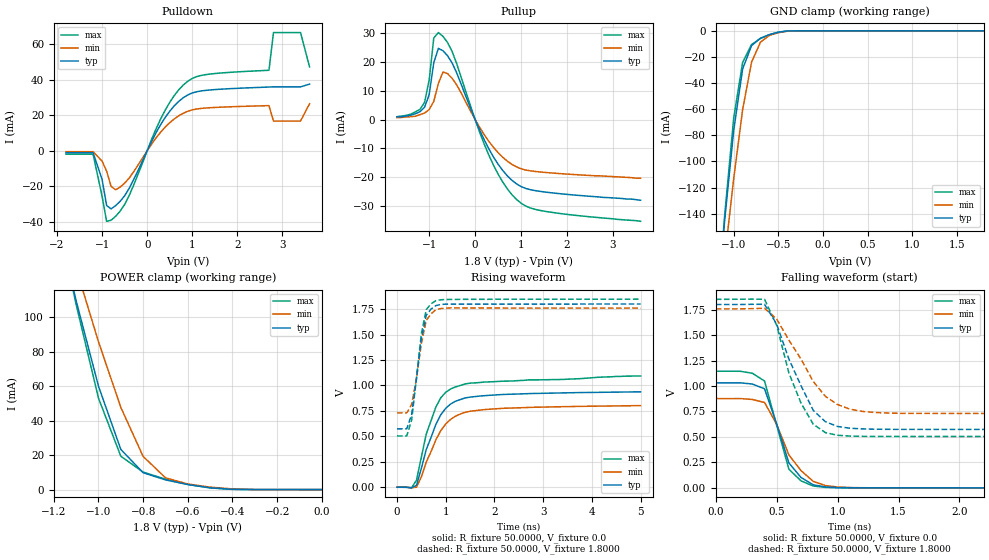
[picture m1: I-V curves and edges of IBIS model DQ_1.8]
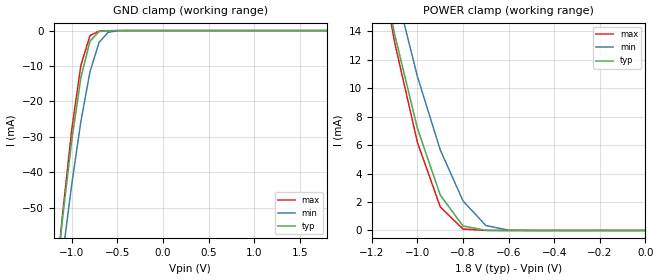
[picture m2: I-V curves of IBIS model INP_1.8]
|*** ISSI Synchronous Sram IBIS Model ***
[IBIS ver]	3.2
[File name]	is61nvvp204836165bga.ibs
[File Rev]	1.0
[Date]	May 13,2013
[Notes]
|--- Version History --------------------------------
|1.0: prelimiary
[Disclaimer]	This information is for modeling purpose only
		and is not guaranteed
[Copyright]	INTEGRATED SILICON SOLUTION, INC. 2011
[Component]	IS61NVVP204836_165BGA
[Manufacturer]	ISSI
[Package]
| variable   typ   min   max
R_pkg		100.34m			23.84m			218.59m
L_pkg		1.3400nH		0.3700nH		3.0300nH
C_pkg		41.410pF		0.4200pF		150.38pF
[Pin]  signal_name   model_name   R_pin   L_pin   C_pin
R11   A   INP_1.8
R10   A   INP_1.8
R9   A   INP_1.8
R8   A   INP_1.8
R7   TCK   INP_1.8
R6   A0   INP_1.8
R5   TMS   INP_1.8
R4   A   INP_1.8
R3   A   INP_1.8
R2   A   INP_1.8
R1   MODE   INP_1.8
P11   NC   NC
P10   A   INP_1.8
P9   A   INP_1.8
P8   A   INP_1.8
P7   TDO   DQ_1.8
P6   A1   INP_1.8
P5   TDI   INP_1.8
P4   A   INP_1.8
P3   A   INP_1.8
P2   A   INP_1.8
P1   NC   NC
N11   DQPa   DQ_1.8
N10   NC   NC
N9   VDDQ   POWER
N8   VSS   GND
N7   NC   NC
N6   NC   NC
N5   NC   NC
N4   VSS   GND
N3   VDDQ   POWER
N2   NC   NC
N1   DQPd   DQ_1.8
M11   DQa   DQ_1.8
M10   DQa   DQ_1.8
M9   VDDQ   POWER
M8   VDD   POWER
M7   VSS   GND
M6   VSS   GND
M5   VSS   GND
M4   VDD   POWER
M3   VDDQ   POWER
M2   DQd   DQ_1.8
M1   DQd   DQ_1.8
L11   DQa   DQ_1.8
L10   DQa   DQ_1.8
L9   VDDQ   POWER
L8   VDD   POWER
L7   VSS   GND
L6   VSS   GND
L5   VSS   GND
L4   VDD   POWER
L3   VDDQ   POWER
L2   DQd   DQ_1.8
L1   DQd   DQ_1.8
K11   DQa   DQ_1.8
K10   DQa   DQ_1.8
K9   VDDQ   POWER
K8   VDD   POWER
K7   VSS   GND
K6   VSS   GND
K5   VSS   GND
K4   VDD   POWER
K3   VDDQ   POWER
K2   DQd   DQ_1.8
K1   DQd   DQ_1.8
J11   DQa   DQ_1.8
J10   DQa   DQ_1.8
J9   VDDQ   POWER
J8   VDD   POWER
J7   VSS   GND
J6   VSS   GND
J5   VSS   GND
J4   VDD   POWER
J3   VDDQ   POWER
J2   DQd   DQ_1.8
J1   DQd   DQ_1.8
H11   ZZ   INP_1.8
H10   NC   NC
H9   NC   NC
H8   VDD   POWER
H7   VSS   GND
H6   VSS   GND
H5   VSS   GND
H4   VDD   POWER
H3   NC   NC
H2   NC   NC
H1   NC   NC
G11   DQb   DQ_1.8
G10   DQb   DQ_1.8
G9   VDDQ   POWER
G8   VDD   POWER
G7   VSS   GND
G6   VSS   GND
G5   VSS   GND
G4   VDD   POWER
G3   VDDQ   POWER
G2   DQc   DQ_1.8
G1   DQc   DQ_1.8
F11   DQb   DQ_1.8
F10   DQb   DQ_1.8
F9   VDDQ   POWER
F8   VDD   POWER
F7   VSS   GND
F6   VSS   GND
F5   VSS   GND
F4   VDD   POWER
F3   VDDQ   POWER
F2   DQc   DQ_1.8
F1   DQc   DQ_1.8
E11   DQb   DQ_1.8
E10   DQb   DQ_1.8
E9   VDDQ   POWER
E8   VDD   POWER
E7   VSS   GND
E6   VSS   GND
E5   VSS   GND
E4   VDD   POWER
E3   VDDQ   POWER
E2   DQc   DQ_1.8
E1   DQc   DQ_1.8
D11   DQb   DQ_1.8
D10   DQb   DQ_1.8
D9   VDDQ   POWER
D8   VDD   POWER
D7   VSS   GND
D6   VSS   GND
D5   VSS   GND
D4   VDD   POWER
D3   VDDQ   POWER
D2   DQc   DQ_1.8
D1   DQc   DQ_1.8
C11   DQPb   DQ_1.8
C10   NC   NC
C9   VDDQ   POWER
C8   VSS   GND
C7   VSS   GND
C6   VSS   GND
C5   VSS   GND
C4   VSS   GND
C3   VDDQ   POWER
C2   NC   NC
C1   DQPc   DQ_1.8
B11   NC   NC
B10   A   INP_1.8
B9   A   INP_1.8
B8   OEB   INP_1.8
B7   WEB   INP_1.8
B6   CLK   INP_1.8
B5   BWaB   INP_1.8
B4   BWdB   INP_1.8
B3   CE2B   INP_1.8
B2   A   INP_1.8
B1   NC   NC
A11   NC   NC
A10   A   INP_1.8
A9   A   INP_1.8
A8   ADV   INP_1.8
A7   CKEB   INP_1.8
A6   CE2B   INP_1.8
A5   BWbB   INP_1.8
A4   BWcB   INP_1.8
A3   CEB   INP_1.8
A2   A   INP_1.8
A1   NC   NC
| Models and submodels in the file (2): DQ_1.8 (3-state), INP_1.8 (Input)
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|   Model DQ_1.8
[Model]		DQ_1.8
Model_type	3-state
Polarity   Non-Inverting
Enable   Active-Low
Vmeas = 	0.7500V
Cref = 		5.0000pF
Rref = 		50.0000
Vref = 		0.8000V
C_comp   3.8290pF   3.3420pF   4.0300pF|
[Temperature Range]	  25.0000   100.0000   0.0
[Voltage Range]   1.8000V   1.7000V   1.9000V
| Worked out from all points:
|   slope of the pulldown table from 0 to 0.27 V, typ, clamps not added: 20.1 ohm
|   slope of the pullup table from 0 to 0.27 V, typ, clamps not added: 29.1 ohm
|   GND clamp passes 1 mA (typ) near -0.49 V on its own axis
|   POWER clamp passes 1 mA (typ) near -0.49 V on its own axis
|   rising waveform, R_fixture 50.0000, V_fixture 0.0: 20-80 % time 458ps typ, 504ps min, 428ps max; typ from 0 V to 0.937 V
|   rising waveform, R_fixture 50.0000, V_fixture 1.8000: 20-80 % time 212ps typ, 215ps min, 202ps max; typ from 0.574 V to 1.8 V
|   falling waveform, R_fixture 50.0000, V_fixture 0.0: 20-80 % time 184ps typ, 232ps min, 159ps max; typ from 1.03 V to 0 V
|   falling waveform, R_fixture 50.0000, V_fixture 1.8000: 20-80 % time 261ps typ, 323ps min, 225ps max; typ from 1.8 V to 0.574 V
[Pulldown]
|Voltage	  I(typ)   I(min)   I(max)
-1.8V     -1.1mA     -531.4uA   -1.933mA
-1.2V     -1.1mA     -531.4uA   -1.933mA
-1V       -16.17mA   -5.85mA    -25.61mA
-900mV    -30.82mA   -11.44mA   -39.73mA
-800mV    -32.74mA   -20.11mA   -39.13mA
-400mV    -21.21mA   -15.41mA   -25.25mA
400mV     18.75mA    13.32mA    22.87mA
900mV     31.42mA    22.22mA    39.13mA
2.7V      35.87mA    25.41mA    45.31mA
2.8V      35.97mA    16.71mA    66.53mA
3.4V      35.97mA    16.71mA    66.53mA
3.6V      37.5mA     26.46mA    47.19mA
[Pullup]
|Voltage	  I(typ)   I(min)   I(max)
-1.7V     900uA      630uA      990uA
-1.3V     2mA        1.134mA    2.662mA
-1.1V     4.3mA      2.25mA     5.962mA
-1V       8.6mA      3.483mA    13.72mA
-900mV    19.73mA    6.273mA    28.28mA
-800mV    24.69mA    12.51mA    30.17mA
-700mV    23.88mA    16.48mA    28.87mA
-500mV    19.6mA     14.29mA    23.58mA
300mV     -10.22mA   -7.61mA    -12.41mA
900mV     -22.31mA   -16.43mA   -27.72mA
1.5V      -25.11mA   -18.32mA   -31.79mA
3.6V      -28mA      -20.34mA   -35.31mA
[GND_clamp]
|Voltage	  I(typ)   I(min)   I(max)
-1.8V     -699.5mA   -630.9mA   -769.6mA
-1.2V     -220.2mA   -237.3mA   -225.5mA
-1.1V     -144.4mA   -173.5mA   -140.5mA
-1V       -76.37mA   -113.2mA   -66.75mA
-900mV    -29.2mA    -60.35mA   -24.21mA
-800mV    -11.34mA   -23.99mA   -10.5mA
-700mV    -5.573mA   -8.7mA     -5.882mA
-600mV    -2.907mA   -3.456mA   -3.007mA
-500mV    -1.075mA   -1.407mA   -999.2uA
-400mV    -173.9uA   -365.4uA   -128uA
1.8V      2.34nA     184.5nA    2.08nA
[POWER_clamp]
|Voltage	  I(typ)   I(min)   I(max)
-1.8V     524.9mA    464.4mA    580.5mA
-1.2V     164.3mA    173.4mA    169.2mA
-1.1V     109.5mA    128.3mA    107.3mA
-1V       59.99mA    85.74mA    53.06mA
-900mV    23.31mA    47.72mA    19.37mA
-800mV    9.803mA    19.24mA    10.14mA
-700mV    5.64mA     6.854mA    6.056mA
-600mV    2.92mA     3.245mA    3.006mA
-500mV    1.061mA    1.426mA    981.4uA
-400mV    183.6uA    396.9uA    135.3uA
0V        2.34nA     17.95nA    3.205nA
[Ramp]
| variable   typ   min   max
dV/dt_r		0.5623/0.4256n   0.4811/0.4247n   0.6354/0.4100n
dV/dt_f		0.7357/0.2222n   0.6457/0.2069n   0.7931/0.2538n
R_load =	50.0000
[Rising Waveform]
R_fixture=	50.0000
V_fixture=	0.0
V_fixture_min=	0.0
V_fixture_max=	0.0
|time   V(typ)   V(min)   V(max)
0s        0V         0V         0V
300ps     -6.035mV   -4.762mV   -4.194mV
400ps     18.96mV    486.8uV    69.03mV
600ps     370.5mV    247mV      521.7mV
800ps     620mV      467.9mV    790.2mV
900ps     712.9mV    557.2mV    879.6mV
1.1ns     817.3mV    666.8mV    965.5mV
1.4ns     877.6mV    736.7mV    1.015V
1.9ns     903.3mV    766.6mV    1.035V
5ns       937.2mV    801.8mV    1.093V
[Rising Waveform]
R_fixture=	50.0000
V_fixture=	1.8000
V_fixture_min=	1.8500
V_fixture_max=	1.7500
|time   V(typ)   V(min)   V(max)
0s        573.8mV    730.3mV    504.1mV
200ps     573.9mV    730.3mV    504.2mV
300ps     713.7mV    812.3mV    659.4mV
400ps     1.067V     1.071V     1.076V
500ps     1.46V      1.412V     1.51V
600ps     1.689V     1.637V     1.745V
700ps     1.752V     1.705V     1.802V
800ps     1.784V     1.744V     1.833V
1.2ns     1.799V     1.762V     1.845V
5ns       1.8V       1.76V      1.848V
[Falling Waveform]
R_fixture=	50.0000
V_fixture=	0.0
V_fixture_min=	0.0
V_fixture_max=	0.0
|time   V(typ)   V(min)   V(max)
0s        1.031V     876.6mV    1.145V
300ps     1.019V     867.6mV    1.125V
400ps     972.5mV    838.1mV    1.049V
500ps     626.1mV    622.4mV    612.9mV
600ps     244.7mV    322.8mV    182.9mV
700ps     101.5mV    168.6mV    68.26mV
800ps     29.89mV    63.85mV    18.06mV
900ps     8.638mV    22.26mV    4.629mV
1.2ns     563.4uV    1.383mV    368.3uV
5ns       26.68uV    38.84uV    22.23uV
[Falling Waveform]
R_fixture=	50.0000
V_fixture=	1.8000
V_fixture_min=	1.8500
V_fixture_max=	1.7500
|time   V(typ)   V(min)   V(max)
0s        1.8V       1.757V     1.851V
400ps     1.802V     1.763V     1.851V
500ps     1.607V     1.657V     1.594V
600ps     1.264V     1.45V      1.127V
700ps     1.002V     1.263V     831.3mV
800ps     760.7mV    1.044V     624.3mV
900ps     649.1mV    898.2mV    542.1mV
1.1ns     585.4mV    772.7mV    508.4mV
1.4ns     574.7mV    734.9mV    504.6mV
5ns       573.8mV    730.3mV    504.2mV
|   Model INP_1.8
[Model]		INP_1.8
Model_type	Input
Polarity   Non-Inverting
Enable   Active-Low
Vinl = 		0.4000V
Vinh = 		1.6000V
C_comp   3.8290pF   3.3420pF   4.0300pF|
[Temperature Range]	  25.0000   100.0000   0.0
[Voltage Range]   1.8000V   1.7000V   1.9000V
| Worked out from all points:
|   GND clamp passes 1 mA (typ) near -0.73 V on its own axis
|   POWER clamp passes 1 mA (typ) near -0.83 V on its own axis
[GND_clamp]
|Voltage	  I(typ)   I(min)   I(max)
-1.8V     -237.3mA   -225.6mA   -256.2mA
-1.2V     -76.89mA   -84.89mA   -78.19mA
-1.1V     -52.83mA   -63.46mA   -51.66mA
-1V       -30.98mA   -43.42mA   -27.92mA
-900mV    -13.28mA   -25.61mA   -9.811mA
-800mV    -2.971mA   -11.61mA   -1.401mA
-700mV    -287uA     -3.303mA   -148.3uA
-600mV    -52.18uA   -480.7uA   -48.72uA
-500mV    -11.21uA   -45.78uA   -9.079uA
-400mV    -777.9nA   -4.481uA   -394.5nA
1.8V      1.69nA     1.724nA    1.796nA
[POWER_clamp]
|Voltage	  I(typ)   I(min)   I(max)
-1.8V     89.26mA    83.96mA    96.39mA
-1.2V     21.9mA     24.63mA    22.02mA
-1.1V     13.77mA    17.21mA    13.19mA
-1V       7.16mA     10.8mA     6.179mA
-900mV    2.488mA    5.659mA    1.649mA
-800mV    312.9uA    2.071mA    100.3uA
-700mV    9.014uA    348.8uA    1.66uA
-600mV    208.4nA    21.46uA    65.15nA
0V        1.69nA     1.088nA    2.855nA
